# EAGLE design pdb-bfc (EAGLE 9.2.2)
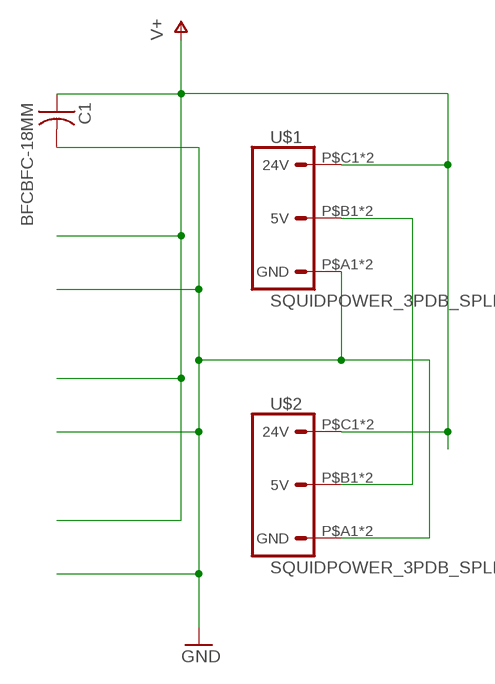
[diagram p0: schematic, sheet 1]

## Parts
C1  BFCBFC-18MM  [BFC-18MM-7-5MM]
U$1  SQUIDPOWER_3PDB_SPLIT  [PDBCONN_3]
U$2  SQUIDPOWER_3PDB_SPLIT  [PDBCONN_3]

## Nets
+5V: U$1.P$B1(5V) U$1.P$B2(5V) U$2.P$B1(5V) U$2.P$B2(5V)
GND: C1.P$1 U$1.P$A1(GND) U$1.P$A2(GND) U$2.P$A1(GND) U$2.P$A2(GND)
V+: C1.P$2 U$1.P$C1(24V) U$1.P$C2(24V) U$2.P$C1(24V) U$2.P$C2(24V)

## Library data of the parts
C1 = power:BFC
U$1 U$2 = connector:SQUIDPOWER_3

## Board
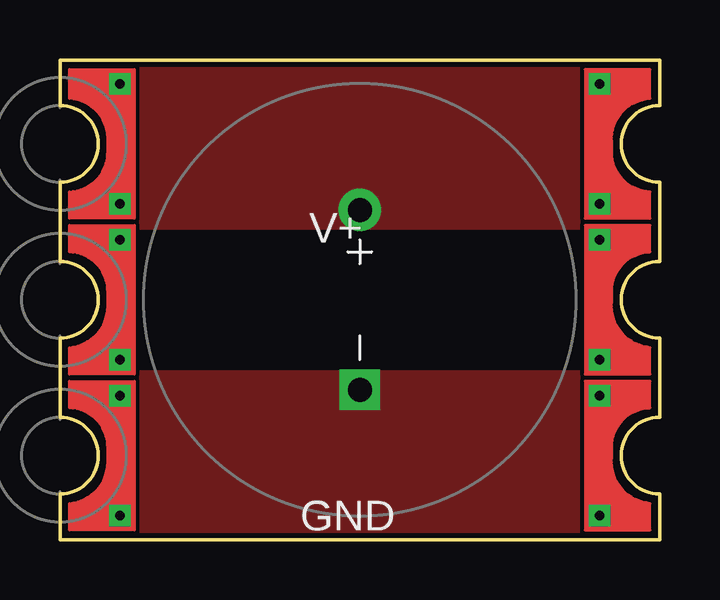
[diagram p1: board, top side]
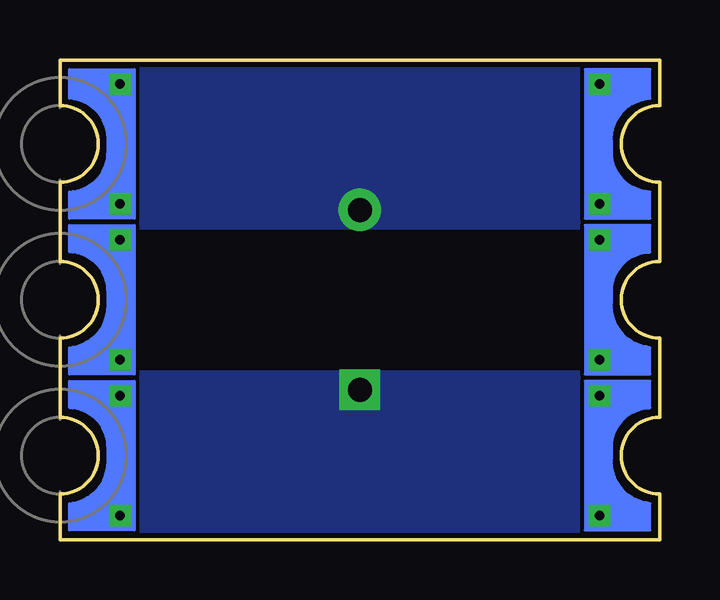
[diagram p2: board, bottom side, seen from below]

Size 25 x 20 mm. Coordinates in mm from the lower left corner, seen from the top.
Outline: 0,5.1 0,8.4 arc90 1.6,10 arc90 0,11.6 0,14.9 arc90 1.6,16.5 arc90 0,18.1 0,20 25,20 25,18.1 arc90 23.4,16.5 arc90 25,14.9 25,11.6 arc90 23.4,10 arc90 25,8.4 25,5.1 arc90 23.4,3.5 arc90 25,1.9 25,0 0,0 0,1.9 arc90 1.6,3.5 arc90 0,5.1
Copper layers (1*16): Top 0.035mm / dielectric 1.5mm / Bottom 0.035mm
Design rules "default *": minimum track width 6mil, minimum drill 0.35mm, track to track 6mil, track to pad 6mil, pad to pad 6mil, via to via 6mil, smd to smd 6mil, copper to edge 8mil, drill to drill 6mil, minimum pad ring 10mil, minimum via ring 8mil, stop-mask expansion 4mil, vias tented up to drill 0mil, thermal gap 10mil

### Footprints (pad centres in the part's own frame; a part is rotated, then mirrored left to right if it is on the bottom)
BFC-18MM-7-5MM = drill 1 pad 1.676 square: P$1 -3.75,0 | drill 1 pad 1.778: P$2 3.75,0
PDBCONN_3 = drill 0.4 square: P$A1 2.5,-9; P$A2 2.5,-4; P$B1 2.5,-2.5; P$B2 2.5,2.5; P$C1 2.5,4; P$C2 2.5,9

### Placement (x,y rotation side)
C1  12.5,10 90 top
U$1  0,10 0 top
U$2  25,10 0 bottom

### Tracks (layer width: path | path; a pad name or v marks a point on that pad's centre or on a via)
+5V
  pour Top (rank 4): -2.5,13 29,13 29,7 -2.5,7
  pour Bottom (rank 4): -3.5,13 30,13 30,7.5 30,7 -3.5,7
GND
  pour Top: -1,7 27.5,7 27.5,-1.5 -1,-1.5
  pour Bottom: -1.5,7 28,7 28,-2 -1.5,-2
V+
  pour Top: -1,13 27.5,13 27.5,21.5 -1,21.5
  pour Bottom: -1.5,13 28,13 28,22 -1.5,22

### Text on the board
tPlace: V+ | GND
